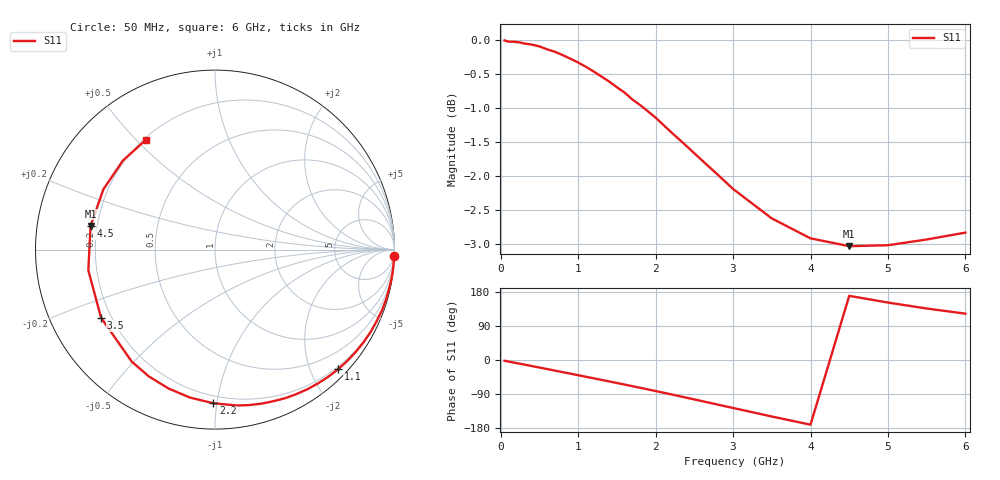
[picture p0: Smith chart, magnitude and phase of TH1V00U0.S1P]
! SIEMENS Discrete & RF Semiconductors
! BAS70
! Si Schottky Diode in SOT23
! VR = 1 V
! S-Parameters:  February  1997
# GHz  S  MA  R  50
!  f  S11
! GHz  MAG  ANG
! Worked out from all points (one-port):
!   34 points, 50 MHz to 6 GHz, reference 50 ohm
!   lowest |S11| = -3.0 dB at 4.5 GHz (marker M1), VSWR 5.80, Z = 8.7 + j4.54 ohm
!   |S11| at or under -10 dB: nowhere
!   S11 on the Smith chart (normalised r, x): 50 MHz: 0, -57; 1.1 GHz: 0.16, -2.45; 2.2 GHz: 0.15, -0.98; 3.5 GHz: 0.16, -0.27; 4.5 GHz: 0.17, +0.09; 6 GHz: 0.21, +0.53
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0.05  1 -2.0
0.1  0.9979 -4.1
0.25  0.9965 -9.9
0.4  0.993 -15.9
0.5  0.9899 -19.9
0.6  0.985 -23.9
0.7  0.981 -28.0
0.8  0.9755 -32.0
0.9  0.9695 -36.0
1.1  0.9563 -44.2
1.2  0.9487 -48.3
1.4  0.9328 -56.5
1.5  0.9238 -60.7
1.6  0.9154 -64.8
1.8  0.8963 -73.3
1.9  0.8869 -77.6
2  0.8774 -81.9
2.2  0.8561 -90.6
2.4  0.8361 -99.6
2.6  0.816 -108.5
2.8  0.7968 -117.6
3  0.7776 -126.6
3.5  0.7397 -149.1
4  0.7151 -170.7
4.5  0.7057 169.3
5  0.7068 151.6
5.5  0.7137 135.9
6  0.7221 122.3
